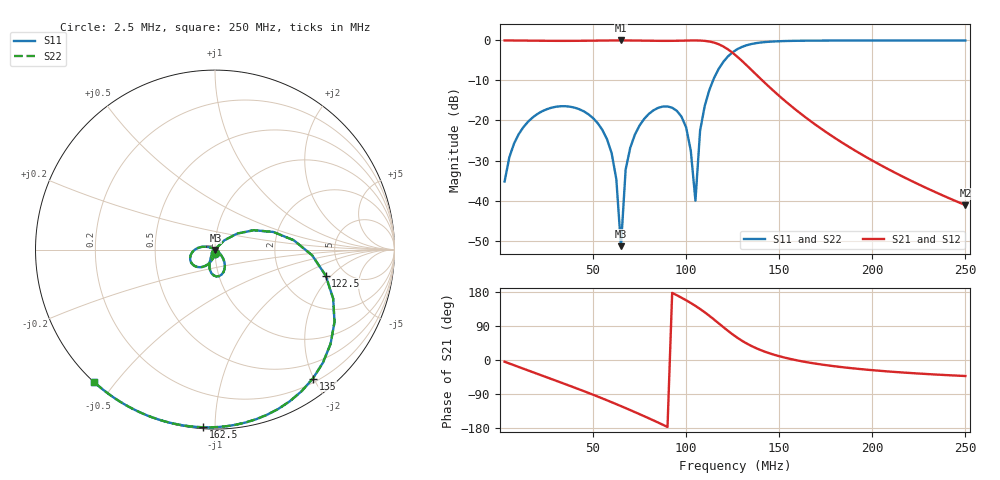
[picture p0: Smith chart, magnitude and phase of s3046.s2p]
!2-port S-parameter file
!Title: test for scattering parameters
!Generated by ngspice at Tue May  9 10:09:54  2023
# Hz S RI R 50
!freq  ReS11  ImS11  ReS21  ImS21  ReS12  ImS12  ReS22  ImS22
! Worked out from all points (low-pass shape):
!   100 points, 2.5 MHz to 250 MHz, reference 50 ohm
!   highest |S21| = 0.00 dB at 65 MHz (marker M1); lowest = -41.2 dB at 250 MHz (marker M2)
!   |S21| within 3 dB of the highest: start of sweep to 124.7 MHz
!   lowest |S11| = -51.4 dB at 65 MHz (marker M3), VSWR 1.01, Z = 50.2 - j0.141 ohm
!   |S11| at or under -10 dB: start of sweep to 114.5 MHz
!   |S22| runs from -51.4 to 0.0 dB; largest |S21 - S12| = 0
!   S11 on the Smith chart (normalised r, x): 2.5 MHz: 1.00, -0.03; 122.5 MHz: 3.57, -1.72; 135 MHz: 0.26, -1.99; 162.5 MHz: 0.01, -0.94; 250 MHz: 0.00, -0.44
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2500000  -0.00136 -0.0173  0.9967 -0.0796  0.9967 -0.0796  -0.00136 -0.0173
7500000  -0.0121 -0.0496  0.9703 -0.2363  0.9703 -0.2363  -0.0121 -0.0496
1.75e7  -0.0574 -0.0924  0.8443 -0.5246  0.8443 -0.5246  -0.0574 -0.0924
4.5e7  -0.129 -0.018  0.1369 -0.982  0.1369 -0.982  -0.129 -0.018
6e7  -0.0363 0.0142  -0.3645 -0.9303  -0.3645 -0.9303  -0.0363 0.0142
6.25e7  -0.0166 0.00828  -0.4462 -0.8947  -0.4462 -0.8947  -0.0166 0.00828
6.5e7  0.00229 -0.0014  -0.5252 -0.851  -0.5252 -0.851  0.00229 -0.0014
6.75e7  0.0194 -0.0146  -0.6005 -0.7993  -0.6005 -0.7993  0.0194 -0.0146
7e7  0.0339 -0.0308  -0.6711 -0.7399  -0.6711 -0.7399  0.0339 -0.0308
8.5e7  0.0369 -0.1391  -0.9566 -0.2533  -0.9566 -0.2533  0.0369 -0.1391
1e8  -0.0312 -0.076  -0.9216 0.3792  -0.9216 0.3792  -0.0312 -0.076
1.025e8  -0.0207 -0.0365  -0.8691 0.4929  -0.8691 0.4929  -0.0207 -0.0365
1.05e8  0.00603 0.00791  -0.7963 0.6048  -0.7963 0.6048  0.00603 0.00791
1.075e8  0.0532 0.0524  -0.7002 0.71  -0.7002 0.71  0.0532 0.0524
1.1e8  0.1234 0.0892  -0.5789 0.801  -0.5789 0.801  0.1234 0.0892
1.225e8  0.6168 -0.1445  0.1764 0.7529  0.1764 0.7529  0.6168 -0.1445
1.275e8  0.6657 -0.4039  0.325 0.5355  0.325 0.5355  0.6657 -0.4039
1.35e8  0.5452 -0.7185  0.3426 0.26  0.3426 0.26  0.5452 -0.7185
1.625e8  -0.0645 -0.99  0.1168 -0.00761  0.1168 -0.00761  -0.0645 -0.99
1.675e8  -0.1382 -0.9847  0.0948 -0.0133  0.0948 -0.0133  -0.1382 -0.9847
2.1e8  -0.5107 -0.8582  0.0203 -0.0121  0.0203 -0.0121  -0.5107 -0.8582
2.5e8  -0.6717 -0.7393  0.00648 -0.00589  0.00648 -0.00589  -0.6717 -0.7393
